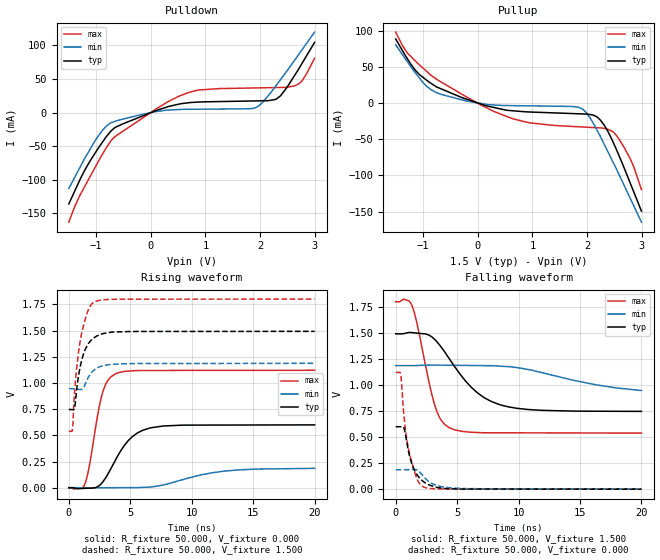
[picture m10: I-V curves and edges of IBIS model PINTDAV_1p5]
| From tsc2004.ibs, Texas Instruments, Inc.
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| Model 1.5 V PINTDAV
[Model]   PINTDAV_1p5
Model_type  Output
Polarity   Non-Inverting
Enable   Active-Low
Vmeas = 0.8
Vref = 0.8
Cref = 15pF
Rref = 50
|   typ   min   max
|   (nom PVT)   (Fast PVT)   (slow PVT)
|   Output High
C_comp   8.83242E-12   8.75145E-12   9.03821E-12
|   Output Low
|C_comp   8.9142E-12   8.63136E-12   8.95536E-12
| Where   nom PVT is  Nominal Process, 3.3V, 25C
|   Fast PVT is Strong Process, 3.6V, -40C
|   Slow PVT is Weak Process, 3.0V, 85C
|C_comp - from L-C Tank method, L = 1nH, peak frequency ~ 1.7GHz
[Voltage Range]   1.5   1.2   1.8
[Temperature Range]   30   88   -40
|Ambient Temperature Range 27   85   -40
[Pullup Reference]   1.5   1.2   1.8
[Pulldown Reference]   0   0   0
[Power Clamp Reference]   1.5   1.2   1.8
[GND Clamp Reference]   0   0   0
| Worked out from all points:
|   slope of the pulldown table from 0 to 0.225 V, typ, clamps not added: 34.2 ohm
|   slope of the pullup table from 0 to 0.225 V, typ, clamps not added: 44.3 ohm
|   falling waveform, R_fixture 50.000, V_fixture 1.500: 20-80 % time 3.16ns typ, 5.48ns min, 1.41ns max; typ from 1.49 V to 0.747 V
|   rising waveform, R_fixture 50.000, V_fixture 0.000: 20-80 % time 1.97ns typ, 3.92ns min, 1.03ns max; typ from 0 V to 0.6 V
|   rising waveform, R_fixture 50.000, V_fixture 1.500: 20-80 % time 836ps typ, 885ps min, 798ps max; typ from 0.747 V to 1.49 V
|   falling waveform, R_fixture 50.000, V_fixture 0.000: 20-80 % time 989ps typ, 1.18ns min, 846ps max; typ from 0.6 V to 0 V
[Pulldown]
|   Voltage   I(typ)   I(min)   I(max)
-1.5V     -136mA     -113mA     -163.3mA
-1.207V   -85.56mA   -68.01mA   -109.7mA
-810.6mV  -35.59mA   -20.03mA   -51.85mA
-649.8mV  -22.01mA   -12.96mA   -35.64mA
82.56mV   2.528mA    1.247mA    4.607mA
506.1mV   12.42mA    4.443mA    24.07mA
864.4mV   15.58mA    4.989mA    33.45mA
1.932V    17.35mA    7.747mA    36.72mA
2.284V    19.61mA    39.42mA    37.24mA
2.374V    25.06mA    49.25mA    37.38mA
2.713V    66.03mA    87.39mA    43.05mA
2.995V    104.5mA    119.9mA    80.97mA
[Pullup]
|   Voltage   I(typ)   I(min)   I(max)
-1.5V     88.94mA    80.86mA    98.51mA
-1.288V   61.82mA    57.62mA    69.72mA
-1.143V   45.79mA    42.35mA    58.72mA
-931.1mV  31.74mA    23.28mA    43.94mA
-687.9mV  20.51mA    12.67mA    30.26mA
145.2mV   -3.379mA   -1.397mA   -5.677mA
634.1mV   -10.42mA   -3.3mA     -21.36mA
1.926V    -14.83mA   -8.455mA   -32.93mA
2.245V    -23.45mA   -46.16mA   -34.22mA
2.518V    -60.88mA   -88.15mA   -42.73mA
2.783V    -109.3mA   -130.6mA   -75.79mA
2.995V    -149.4mA   -164.7mA   -119.4mA
[Ramp]
R_load = 50
|   typ   min   max
dV/dt_r   0.360026/1.9655e-009   0.110786/3.86162e-009  0.672478/1.02773e-009
dV/dt_f   0.452939/3.14478e-009   0.15393/5.41753e-009  0.756907/1.40757e-009
[Falling Waveform]
R_fixture = 50.000
V_fixture = 1.500
V_fixture_min = 1.200
V_fixture_max = 1.800
C_fixture = 0.000
|  time   V(typ)   V(min)   V(max)
0s        1.492V     1.187V     1.8V
654.4ps   1.494V     1.187V     1.826V
1.325ns   1.503V     1.187V     1.763V
1.728ns   1.499V     1.188V     1.595V
3.175ns   1.438V     1.192V     808.7mV
3.697ns   1.365V     1.191V     663mV
4.357ns   1.254V     1.19V      590.7mV
6.258ns   966.4mV    1.188V     546.2mV
8.683ns   804.4mV    1.18V      541.4mV
20ns      747.1mV    947.6mV    538.5mV
[Rising Waveform]
R_fixture = 50.000
V_fixture = 0.000
V_fixture_min = 0.000
V_fixture_max = 0.000
C_fixture = 0.000
|  time   V(typ)   V(min)   V(max)
0s        108.1nV    2.698mV    11.14nV
1.301ns   -5.193mV   166.5uV    34.81mV
1.607ns   -4.07mV    -427.4uV   169.4mV
2.72ns    49.15mV    146.7uV    895.3mV
3.175ns   130mV      459.6uV    1.024V
3.809ns   267.5mV    895.2uV    1.088V
5.174ns   488.2mV    1.832mV    1.116V
6.695ns   572.8mV    8.159mV    1.119V
12.5ns    598.4mV    156.9mV    1.12V
20ns      600mV      185.6mV    1.121V
[Rising Waveform]
R_fixture = 50.000
V_fixture = 1.500
V_fixture_min = 1.200
V_fixture_max = 1.800
C_fixture = 0.000
|  time   V(typ)   V(min)   V(max)
0s        747.1mV    947.6mV    538.5mV
299.8ps   745.5mV    944.3mV    559.5mV
463.8ps   760.6mV    942.4mV    902.2mV
594.3ps   887.6mV    941mV      1.086V
787ps     1.063V     938.9mV    1.291V
1.016ns   1.2V       937.9mV    1.457V
1.586ns   1.374V     1.053V     1.698V
2.107ns   1.435V     1.128V     1.776V
4.324ns   1.488V     1.183V     1.799V
20ns      1.492V     1.187V     1.8V
[Falling Waveform]
R_fixture = 50.000
V_fixture = 0.000
V_fixture_min = 0.000
V_fixture_max = 0.000
C_fixture = 0.000
|  time   V(typ)   V(min)   V(max)
0s        600mV      185.6mV    1.121V
405.7ps   600mV      186.4mV    1.102V
621.9ps   600.6mV    186.8mV    773.4mV
756.8ps   549.1mV    187mV      612.3mV
1.167ns   302.5mV    187.8mV    321.2mV
1.758ns   133.8mV    183.4mV    91.62mV
2.272ns   71.6mV     121.5mV    21mV
3.239ns   19.51mV    39.82mV    4.205mV
4.635ns   3.477mV    11.01mV    1.061mV
20ns      108.2nV    2.698mV    8.308nV
